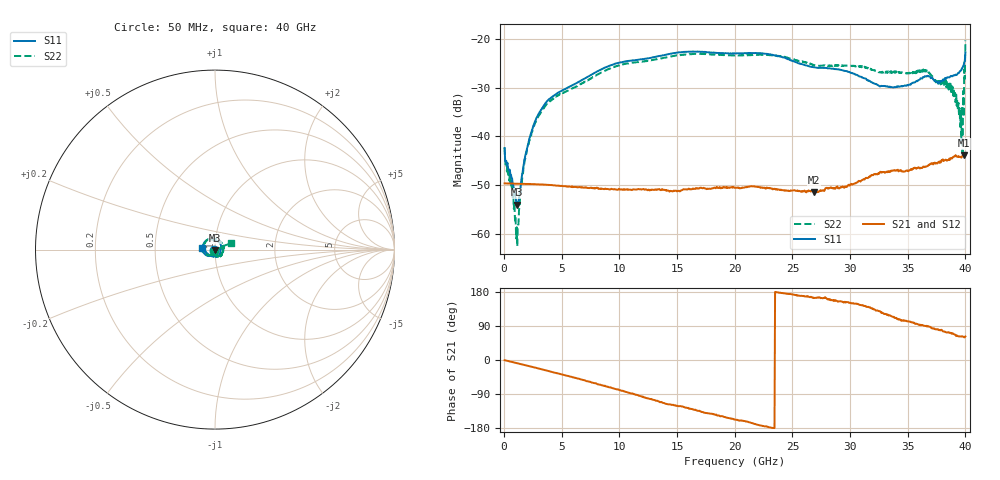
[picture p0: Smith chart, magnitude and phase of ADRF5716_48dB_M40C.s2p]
! Device: ADRF5716
! Description: 30GHz 2-Bit Digital Attenuator
! Frequency: 100 MHz – 30 GHz
! Ports:
! ATTIN  = Port 1
! ATTOUT = Port 2
! State: 48 dB Attenuation selected
! Supply Voltage:
! VDD  =  +3.30 Volts
! VSS  =  -3.30 Volts
! Control Voltages:
! D5 = 3.3V, D6 = 3.3V
! Temperature = -40 C
! Data: Data was collected using a calibrated network analyzer.
!  The reference plane is the package pins of ADRF5716 switch.
! Note: Analog Devices supplies this data as a sample of measured data for this product.
!  Your particular data for this product may vary.
!  Analog Devices reserves the right to change this data at anytime
# HZ S DB R 50
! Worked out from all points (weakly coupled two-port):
!   800 points, 50 MHz to 40 GHz, reference 50 ohm
!   highest |S21| = -43.86 dB at 39.85 GHz (marker M1); lowest = -51.5 dB at 26.9 GHz (marker M2)
!   lowest |S11| = -54.0 dB at 1.15 GHz (marker M3), VSWR 1.00, Z = 49.9 - j0.147 ohm
!   |S11| at or under -10 dB: start of sweep to end of sweep
!   |S22| runs from -62.5 to -20.3 dB; largest |S21 - S12| = 0
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5e7  -42.42 -138.7  -49.66 -0.7  -49.66 -0.7  -42.29 -136.6
6e8  -47.88 176.9  -49.69 -4.6  -49.69 -4.6  -48.99 169.4
9.5e8  -52.27 -163.3  -49.71 -7.2  -49.71 -7.2  -57.29 177.2
1.15e9  -54.01 -132.4  -49.72 -8.7  -49.72 -8.7  -62.55 -111.6
1.8e9  -44.47 -81.3  -49.77 -13.4  -49.77 -13.4  -44.56 -70.8
2.8e9  -36.27 -87.5  -49.86 -20.9  -49.86 -20.9  -36.66 -83.6
3.9e9  -32.38 -103.2  -49.99 -29.4  -49.99 -29.4  -32.96 -102.2
6.75e9  -28.43 -122.4  -50.43 -51.9  -50.43 -51.9  -29.18 -124.5
9.65e9  -25.08 -141.4  -50.90 -76.7  -50.90 -76.7  -25.63 -144.4
1.34e10  -23.52 -164.2  -50.88 -109.3  -50.88 -109.3  -24.09 -170.1
2.005e10  -22.97 152.1  -50.57 -157.2  -50.57 -157.2  -23.35 142.0
2.305e10  -23.17 127.2  -50.58 -177.8  -50.58 -177.8  -23.36 116.8
2.67e10  -25.76 95.4  -51.13 165.1  -51.13 165.1  -25.28 77.7
2.69e10  -25.84 94.0  -51.50 163.6  -51.50 163.6  -25.44 76.2
3.335e10  -29.80 -2.1  -47.25 117.3  -47.25 117.3  -26.89 -5.7
3.655e10  -27.70 -65.7  -46.25 89.5  -46.25 89.5  -26.36 -52.0
3.83e10  -28.16 -106.0  -44.77 73.7  -44.77 73.7  -28.46 -76.8
3.91e10  -27.47 -131.0  -44.12 66.4  -44.12 66.4  -31.09 -80.1
3.955e10  -26.64 -149.1  -44.25 62.3  -44.25 62.3  -38.09 -92.7
3.975e10  -25.96 -160.4  -44.07 62.5  -44.07 62.5  -43.35 -27.0
3.985e10  -25.47 -167.7  -43.86 60.7  -43.86 60.7  -36.00 15.7
4e10  -22.79 174.1  -43.87 62.1  -43.87 62.1  -20.32 21.0
